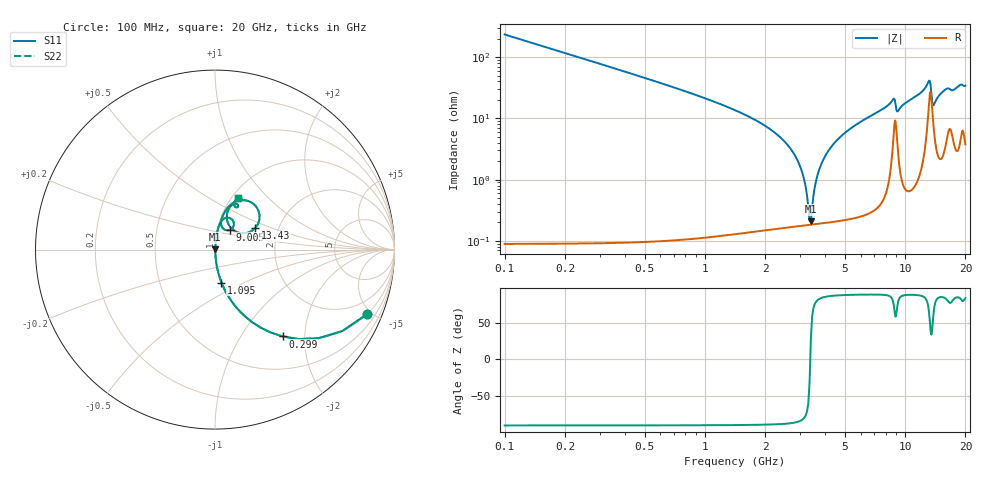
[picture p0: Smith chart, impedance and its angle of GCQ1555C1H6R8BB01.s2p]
!Murata Part Number: GCQ1555C1H6R8BB01
!These Parameters are Measured in Series Mode Connection
!Data Generated on Mar 13, 2026
!  o--ll--o
!Port1  Port2
!  o------o
!Operation Temp=25[degC], DC Bias Voltage=0[V]
!Freq. Start=100[MHz] Stop=20[GHz] 401[Steps]
# Hz S RI R 50
!Freq.(Hz) S11(Real) S11(Imag) S21(Real) S21(Imag) S12(Real) S12(Imag) S22(Real) S22(Imag)
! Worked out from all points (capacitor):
!   401 points, 100 MHz to 20 GHz, reference 50 ohm
!   read as one part in series: C = 6.8 pF near 199.5 MHz
!   lowest |Z| = 208 mohm at 3.384 GHz (marker M1)
!   series resonance near 3.36 GHz, so ESL is about 330 pH
!   S11 on the Smith chart (normalised r, x): 100 MHz: 1.00, -4.68; 299 MHz: 1.00, -1.55; 1.095 GHz: 1.00, -0.38; 9.005 GHz: 1.15, +0.26; 13.43 GHz: 1.52, +0.39; 20 GHz: 1.08, +0.68
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1e8  0.8453 -0.3614  0.1547 0.3614  0.1547 0.3614  0.8453 -0.3614
2.99e8  0.3763 -0.4839  0.6237 0.4839  0.6237 0.4839  0.3763 -0.4839
5.975e8  0.1264 -0.331  0.8736 0.331  0.8736 0.331  0.1264 -0.331
1.095e9  0.0362 -0.1838  0.9638 0.1838  0.9638 0.1838  0.0362 -0.1838
2.73675e9  0.00251 -0.0287  0.9975 0.0287  0.9975 0.0287  0.00251 -0.0287
3.03525e9  0.00196 -0.0142  0.998 0.0142  0.998 0.0142  0.00196 -0.0142
3.284e9  0.00182 -0.00318  0.9982 0.00318  0.9982 0.00318  0.00182 -0.00318
3.3835e9  0.00183 0.000973  0.9982 -0.000973  0.9982 -0.000973  0.00183 0.000973
3.43325e9  0.00185 0.00301  0.9981 -0.00301  0.9981 -0.00301  0.00185 0.00301
3.73175e9  0.00212 0.0147  0.9979 -0.0147  0.9979 -0.0147  0.00212 0.0147
4.22925e9  0.00306 0.0325  0.9969 -0.0325  0.9969 -0.0325  0.00306 0.0325
6.7665e9  0.0149 0.1086  0.9851 -0.1086  0.9851 -0.1086  0.0149 0.1086
8.70675e9  0.0726 0.1779  0.9274 -0.1779  0.9274 -0.1779  0.0726 0.1779
9.00525e9  0.0836 0.1095  0.9164 -0.1095  0.9164 -0.1095  0.0836 0.1095
1.005e10  0.0371 0.1707  0.9629 -0.1707  0.9629 -0.1707  0.0371 0.1707
1.288575e10  0.156 0.2757  0.844 -0.2757  0.844 -0.2757  0.156 0.2757
1.338325e10  0.2391 0.1417  0.7609 -0.1417  0.7609 -0.1417  0.2391 0.1417
1.3433e10  0.2239 0.1197  0.7761 -0.1197  0.7761 -0.1197  0.2239 0.1197
1.3831e10  0.0907 0.1191  0.9093 -0.1191  0.9093 -0.1191  0.0907 0.1191
1.51245e10  0.0788 0.2301  0.9212 -0.2301  0.9212 -0.2301  0.0788 0.2301
1.67165e10  0.1287 0.2392  0.8713 -0.2392  0.8713 -0.2392  0.1287 0.2392
2e10  0.1298 0.2852  0.8702 -0.2852  0.8702 -0.2852  0.1298 0.2852
